|   IBIS model for TI tms320c6670 DSP
[IBIS Ver]   5.0
[Disclaimer]   Please be aware that in the absence of a written agreement
|   Texas Instruments(TI) assumes no liability for:
|   (1) The accuracy of the IBIS models provided to your company,
|   however, the IBIS model is compliant to industry standard
|   IQ Level 2a.  Refer to IBIS Quality Section below for
|   for full details.
|   (2) The proper functioning of these Models in your design
|   or for any resulting applications
|   (3) Infringement of patents, copyrights or intellectual
|   property rights resulting from your use of these
|   models.
|   TI provides IBIS Models as a service to our customers and
|   therefore reserves the right to limit distribution of the
|   Models.  The information is subject to change without notice.
[File Name]  tms320c6670_r1p11.ibs
[File Rev]   1.11
[Date]   16Feb2012
[Source]   Texas Instruments Incorporated
[Copyright]   Property of Texas Instruments Incorporated.
|   Unauthorized reproduction and/or distribution is strictly.
|   prohibited.
|   This product is protected under copyright law and trade
|   secret law as an unpublished work.
|   Created 2010,(C) Copyright 1999-2010,
|   Texas Instruments Incorporated., All Rights Reserved.
|   These commodities are under the U.S. Government
|   distribution license control. As such,they are not to be
|   re-exported without the prior approval of the U.S.
|   Department of Commerce.
[Notes]
   For SerDes simulations use Texas Instruments IBIS AMI models
   Some IV curves contain Non monotonic data points.
|   Model Generated by R.L.L.
|   **For SerDes simulations use Texas Instruments IBIS AMI models**
| Definitions:
|   NT   No termination
|   HT_TH_8mA   Half Termination Thevenin  [50 ohm] [100ohm to Vtt]
|   FT_TH_8mA   Full Termination Thevenin  [50 ohm] [50ohm to Vtt]
|   HT_TH_9mA   Half Termination Thevenin  [45 ohm] [90ohm to Vtt]
|   FT_TH_9mA   Full Termination Thevenin  [45 ohm] [45ohm to Vtt]
|   HT_TH_10mA   Half Termination Thevenin  [40 ohm] [80ohm to Vtt]
|   FT_TH_10mA   Full Termination Thevenin  [40 ohm] [40ohm to Vtt]
| Slew Rate Definitions:
| The Driver Slew Rate is defined by the value of the slew rate pins
|   DDRSLRATE1  DDRSLRATE0
|   FASTEST Slew Rate :   SR1 0;   SR0 0
|   FAST Slew Rate   :   SR1 0;   SR0 1
|   SLOW Slew Rate   :   SR1 1;   SR0 0
|   SLOWEST Slew Rate :   SR1 1;   SR0 1
| To choose the correct model, determine the settings of the DDRSLRATE[1:0] pins.
| Look for the keyword from the tables above to select the proper models.  For
| example; with the recommended 45.3ohm resistor connected to the PTV15 pin the
| drive strength of 9ma would be obtained "9MA_FT9MA". If the DDRSLRATE1 pin is
| pulled high and the DDRSLRATE0 pin is pulled low the slew rate (from the table
| above) would be "SLOW".  For this example the model needed for the address and
| control pins would be CSCDVG_SLOW_9MA, the data and DQM pins would be
| CSCDVG_SLOW_9MA_FT9MA and the DQS pins would be CSCDDVG_SLOW_9MA_FT9MA_N and
| CSCDDVG_SLOW_9MA_FT9MA_P.
|   Revision History
|   GERNERAL COMMENT: All IBIS Quality Notes below reflect latest release
|   and version of IBIS File
|   Revision 1.11 --16Feb 2012
|   -Corrected slew rate settings for fast and slow
|   -Added additional comments in the notes section
|   Revision 1.10 --14Oct 2011
|   -Updated model selectors
|   Revision 1.9 --12Oct 2011
|   -Corrected ACC_OUT & CLK_OUT descriptions
|   Revision 1.8 --29Sept 2011
|   -Corrected cell call error, removed Diff conflicting cells
|   Revision 1.7 --22Sept 2011
|   -Added submodels for bshtltcscddvg and bshtltcscdvg
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[Component] tms320c6670
[Manufacturer] Texas Instruments
[Package Model] 6670
[Package]
|Variable   Typ   Min   Max
R_pkg   1.0013   0.15483   2.0653
L_pkg   2.89689nH  0.94768nH   5.3815nH
C_pkg   1.63791pF  0.87102pF   2.5609pF
[Pin]   signal_name   model_name
A1   VSS   GND   |   GND
A10   DDRDQM4   DM   |   bshtltcscdvg
A11   DVDD15   POWER   |   POWER
A12   DDRCLKOUTP0   CLK_OUT   |   bshtltcscdvg
A13   DDRBA0   ACC_OUT   |   bshtltcscdvg
A14   DDRA00   ACC_OUT   |   bshtltcscdvg
A15   DDRA04   ACC_OUT   |   bshtltcscdvg
A16   DDRCLKOUTP1   CLK_OUT   |   bshtltcscdvg
A17   DVDD15   POWER   |   POWER
A18   DDRCB07   DQ   |   bshtltcscdvg
A19   DDRDQS8P   DQS   |   bshtltcscddvg
A2   DVDD15   POWER   |   POWER
A20   DDRDQM8   DM   |   bshtltcscdvg
A21   DDRDQS3P   DQS   |   bshtltcscddvg
A22   DDRDQM3   DM   |   bshtltcscdvg
A23   DDRD20   DQ   |   bshtltcscdvg
A24   DDRDQS2P   DQS   |   bshtltcscddvg
A25   DDRDQM2   DM   |   bshtltcscdvg
A26   DDRD15   DQ   |   bshtltcscdvg
A27   DDRDQS1P   DQS   |   bshtltcscddvg
A28   DVDD15   POWER   |   POWER
A29   VSS   GND   |   GND
A3   DDRDQS6N   DQS   |   bshtltcscddvg
A4   DDRD51   DQ   |   bshtltcscdvg
A5   DDRD49   DQ   |   bshtltcscdvg
A6   DDRDQS5N   DQS   |   bshtltcscddvg
A7   DDRD40   DQ   |   bshtltcscd
A8   DDRDQM5   DM   |   bshtltcscdvg
A9   DDRDQS4P   DQS   |   bshtltcscddvg
AA1   MCMTXPMDAT   bc1850cghypbfb   |   bc1850cghypbfb
AA10   CVDD   POWER   |   POWER
AA11   VSS   GND   |   GND
AA12   CVDD   POWER   |   POWER
AA13   VSS   GND   |   GND
AA14   CVDD   POWER   |   POWER
AA15   VSS   GND   |   GND
AA16   CVDD   POWER   |   POWER
AA17   VSS   GND   |   GND
AA18   CVDD   POWER   |   POWER
AA19   VSS   GND   |   GND
AA2   MCMTXPMCLK   bc1850cghypbfb   |   bc1850cghypbfb
AA20   CVDD   POWER   |   POWER
AA21   VSS   GND   |   GND
AA22   CVDD   POWER   |   POWER
AA23   VSS   GND   |   GND
AA24   RSV18   NC   |   NC
AA25   VSS   GND   |   GND
AA26   SYSCLKOUT   bc1850cghypbfb   |   bc1850cghypbfb
AA27   RADSYNC   bc1850cghypbfb   |   bc1850cghypbfb
AA28   RP1CLKN   ilvds18g   |   ilvds18g
AA29   RP1FBN   ilvds18g   |   ilvds18g
AA3   MCMRXPMCLK   bc1850cghypbfb   |   bc1850cghypbfb
AA4   VCNTL2   bi2c18gfz   |   bi2c18gfz
AA5   VSS   GND   |   GND
AA6   VSS   GND   |   GND
AA7   VSS   GND   |   GND
AA8   CVDD   POWER   |   POWER
AA9   VSS   GND   |   GND
AB1   VCNTL3   bi2c18gfz   |   bi2c18gfz
AB10   VSS   GND   |   GND
AB11   VSS   GND   |   GND
AB12   VSS   GND   |   GND
AB13   VSS   GND   |   GND
AB14   VSS   GND   |   GND
AB15   AVDDA3   POWER   |   POWER
AB16   VSS   GND   |   GND
AB17   DVDD18   POWER   |   POWER
AB18   VSS   GND   |   GND
AB19   DVDD18   POWER   |   POWER
AB2   VSS   GND   |   GND
AB20   VSS   GND   |   GND
AB21   DVDD18   POWER   |   POWER
AB22   VSS   GND   |   GND
AB23   CVDD   POWER   |   POWER
AB24   VSS   GND   |   GND
AB25   CORECLKSEL   bc1850cghypbfb   |   bc1850cghypbfb
AB26   RSV20   NC   |   NC
AB27   PHYSYNC   bc1850cghypbfb   |   bc1850cghypbfb
AB28   ALTCORECLKN   iclkrx10g   |   iclkrx10g
AB29   ALTCORECLKP   iclkrx10g   |   iclkrx10g
AB3   VCNTL1   bi2c18gfz   |   bi2c18gfz
AB4   VCNTL0   bi2c18gfz   |   bi2c18gfz
AB5   DVDD18   POWER   |   POWER
AB6   VSS   GND   |   GND
AB7   VSS   GND   |   GND
AB8   VSS   GND   |   GND
AB9   VSS   GND   |   GND
AC1   VSS   GND   |   GND
AC10   VDDT2   POWER   |   POWER
AC11   VSS   GND   |   GND
AC12   VDDT2   POWER   |   POWER
AC13   VSS   GND   |   GND
AC14   VDDT2   POWER   |   POWER
AC15   VSS   GND   |   GND
AC16   CORESEL1   bc1850cghypbfb   |   bc1850cghypbfb
AC17   SCL   bi2c18gfz   |   bi2c18gfz
AC18   HOUT   bc1840dghypbfb   |   bc1840dghypbfb
AC19   PORz   ihhv18g   |   RESET
AC2   DVDD18   POWER   |   POWER
AC20   LRESETNMIENz   bc1850cghypbfb   |   bc1850cghypbfb
AC21   BOOTCOMPLETE   bc1850cghypbfb   |   bc1850cghypbfb
AC22   RSV13   NC   |   NC
AC23   RSV03   NC   |   NC
AC24   RESETz   ic18ghypbfb   |   ic18ghypbfb
AC25   NMIz   bc1850cghypbfb   |   bc1850cghypbfb
AC26   TMS   ic18ghypbfb   |   ic18ghypbfb
AC27   TDO   bc1840dghypbfb   |   bc1840dghypbfb
AC28   SYSCLKN   iclkrx10g   |   iclkrx10g
AC29   SYSCLKP   iclkrx10g   |   iclkrx10g
AC3   VSS   GND   |   GND
AC4   DVDD18   POWER   |   POWER
AC5   VSS   GND   |   GND
AC6   VDDT2   POWER   |   POWER
AC7   VSS   GND   |   GND
AC8   VDDT2   POWER   |   POWER
AC9   VSS   GND   |   GND
AD1   CVDD1   POWER   |   POWER
AD10   VSS   GND   |   GND
AD11   VDDT2   POWER   |   POWER
AD12   VSS   GND   |   GND
AD13   VDDT2   POWER   |   POWER
AD14   VSS   GND   |   GND
AD15   CORESEL2   bc1850cghypbfb   |   bc1850cghypbfb
AD16   RSV23   NC   |   NC
AD17   SDA   bi2c18gfz   |   bi2c18gfz
AD18   RESETSTATz   bc1850cghypbfb   |   bc1850cghypbfb
AD19   GPIO02   bc1840dghypbfb   |   bc1840dghypbfb
AD2   VSS   GND   |   GND
AD20   GPIO11   bc1840dghypbfb   |   bc1840dghypbfb
AD21   GPIO15   bc1840dghypbfb   |   bc1840dghypbfb
AD22   RSV12   NC   |   NC
AD23   PACLKSEL   bc1840dghypbfb   |   bc1840dghypbfb
AD24   VSS   GND   |   GND
AD25   EMU05   bc1840dghypbfb   |   bc1840dghypbfb
AD26   TRSTz   ic18ghypbfb   |   ic18ghypbfb
AD27   VSS   GND   |   GND
AD28   TDI   ic18ghypbfb   |   ic18ghypbfb
AD29   TCK   ic18ghypbfb   |   ic18ghypbfb
AD3   CVDD1   POWER   |   POWER
AD4   VSS   GND   |   GND
AD5   VDDT2   POWER   |   POWER
AD6   VSS   GND   |   GND
AD7   VDDT2   POWER   |   POWER
AD8   VSS   GND   |   GND
AD9   VDDT2   POWER   |   POWER
AE1   VSS   GND   |   GND
AE10   VDDT2   POWER   |   POWER
AE11   VDDR4   POWER   |   POWER
AE12   VDDT2   POWER   |   POWER
AE13   VSS   GND   |   GND
AE14   RSV16   NC   |   NC
AE15   VDDR2   POWER   |   POWER
AE16   RSV22   NC   |   NC
AE17   EXTFRAMEEVENT   bc1850cghypbfb   |   bc1850cghypbfb
AE18   GPIO05   bc1840dghypbfb   |   bc1840dghypbfb
AE19   GPIO03   bc1840dghypbfb   |   bc1840dghypbfb
AE2   CVDD1   POWER   |   POWER
AE20   GPIO12   bc1840dghypbfb   |   bc1840dghypbfb
AE21   GPIO09   bc1840dghypbfb   |   bc1840dghypbfb
AE22   LRESETz   bc1850cghypbfb   |   bc1850cghypbfb
AE23   RESETFULLz   ic18ghypbfb   |   ic18ghypbfb
AE24   DVDD18   POWER   |   POWER
AE25   EMU07   bc1840dghypbfb   |   bc1840dghypbfb
AE26   EMU04   bc1840dghypbfb   |   bc1840dghypbfb
AE27   DVDD18   POWER   |   POWER
AE28   EMU02   bc1840dghypbfb   |   bc1840dghypbfb
AE29   EMU00   bc1840dghypbfb   |   bc1840dghypbfb
AE3   VSS   GND   |   GND
AE4   VDDT2   POWER   |   POWER
AE5   RSV17   NC   |   NC
AE6   VDDR3   POWER   |   POWER
AE7   VSS   GND   |   GND
AE8   RSV15   NC   |   NC
AE9   VSS   GND   |   GND
AF1   CVDD1   POWER   |   POWER
AF10   RIOTXP1   NC   |   NC
AF11   VSS   GND   |   GND
AF12   PCIETXN1   NC   |   NC
AF13   PCIETXP1   NC   |   NC
AF14   VSS   GND   |   GND
AF15   VSS   GND   |   GND
AF16   MDCLK   bc1840dghypbfb   |   bc1840dghypbfb
AF17   RSV25   NC   |   NC
AF18   GPIO04   bc1840dghypbfb   |   bc1840dghypbfb
AF19   DVDD18   POWER   |   POWER
AF2   VSS   GND   |   GND
AF20   VSS   GND   |   GND
AF21   GPIO13   bc1840dghypbfb   |   bc1840dghypbfb
AF22   DVDD18   POWER   |   POWER
AF23   TIMO1   bc1850cghypbfb   |   bc1850cghypbfb
AF24   UARTRXD   bc1850cghypbfb   |   bc1850cghypbfb
AF25   EMU06   bc1840dghypbfb   |   bc1840dghypbfb
AF26   EMU10   bc1840dghypbfb   |   bc1840dghypbfb
AF27   EMU08   bc1840dghypbfb   |   bc1840dghypbfb
AF28   EMU03   bc1840dghypbfb   |   bc1840dghypbfb
AF29   EMU01   bc1840dghypbfb   |   bc1840dghypbfb
AF3   SGMII0TXN   NC   |   NC
AF4   SGMII0TXP   NC   |   NC
AF5   VSS   GND   |   GND
AF6   RIOTXN3   NC   |   NC
AF7   RIOTXP3   NC   |   NC
AF8   VSS   GND   |   GND
AF9   RIOTXN1   NC   |   NC
AG1   VSS   GND   |   GND
AG10   RIOTXP0   NC   |   NC
AG11   RIOTXN0   NC   |   NC
AG12   VSS   GND   |   GND
AG13   PCIETXP0   NC   |   NC
AG14   PCIETXN0   NC   |   NC
AG15   VSS   GND   |   GND
AG16   MDIO   bc1850cghypbfb   |   bc1850cghypbfb
AG17   RSV24   NC   |   NC
AG18   GPIO01   bc1840dghypbfb   |   bc1840dghypbfb
AG19   GPIO10   bc1840dghypbfb   |   bc1840dghypbfb
AG2   CVDD1   POWER   |   POWER
AG20   GPIO06   bc1840dghypbfb   |   bc1840dghypbfb
AG21   SPICLK   bc1850cghypbfb   |   bc1850cghypbfb
AG22   VSS   GND   |   GND
AG23   TIMI1   bc1850cghypbfb   |   bc1850cghypbfb
AG24   UARTRTS   bc1850cghypbfb   |   bc1850cghypbfb
AG25   EMU13   bc1840dghypbfb   |   bc1840dghypbfb
AG26   VSS   GND   |   GND
AG27   EMU12   bc1840dghypbfb   |   bc1840dghypbfb
AG28   EMU11   bc1840dghypbfb   |   bc1840dghypbfb
AG29   EMU09   bc1840dghypbfb   |   bc1840dghypbfb
AG3   VSS   GND   |   GND
AG4   SGMII1TXN   NC   |   NC
AG5   SGMII1TXP   NC   |   NC
AG6   VSS   GND   |   GND
AG7   RIOTXN2   NC   |   NC
AG8   RIOTXP2   NC   |   NC
AG9   VSS   GND   |   GND
AH1   CVDD1   POWER   |   POWER
AH10   RIORXN1   NC   |   NC
AH11   VSS   GND   |   GND
AH12   PCIERXN1   NC   |   NC
AH13   PCIERXP1   NC   |   NC
AH14   VSS   GND   |   GND
AH15   CORESEL0   bc1850cghypbfb   |   bc1850cghypbfb
AH16   SRIOSGMIICLKN   iclkrx10g   |   iclkrx10g
AH17   PCIECLKP   iclkrx10g   |   iclkrx10g
AH18   PASSCLKN   iclkrx10g   |   iclkrx10g
AH19   GPIO07   bc1840dghypbfb   |   bc1840dghypbfb
AH2   VSS   GND   |   GND
AH20   GPIO14   bc1840dghypbfb   |   bc1840dghypbfb
AH21   SPISCS0   bc1850cghypbfb   |   bc1850cghypbfb
AH22   SPIDIN   bc1850cghypbfb   |   bc1850cghypbfb
AH23   TIMO0   bc1850cghypbfb   |   bc1850cghypbfb
AH24   UARTCTS   bc1850cghypbfb   |   bc1850cghypbfb
AH25   EMU18   bc1840dghypbfb   |   bc1840dghypbfb
AH26   DVDD18   POWER   |   POWER
AH27   EMU16   bc1840dghypbfb   |   bc1840dghypbfb
AH28   EMU14   bc1840dghypbfb   |   bc1840dghypbfb
AH29   DVDD18   POWER   |   POWER
AH3   SGMII0RXN   NC   |   NC
AH4   SGMII0RXP   NC   |   NC
AH5   VSS   GND   |   GND
AH6   RIORXN3   NC   |   NC
AH7   RIORXP3   NC   |   NC
AH8   VSS   GND   |   GND
AH9   RIORXP1   NC   |   NC
AJ1   VSS   GND   |   GND
AJ10   RIORXP0   NC   |   NC
AJ11   RIORXN0   NC   |   NC
AJ12   VSS   GND   |   GND
AJ13   PCIERXP0   NC   |   NC
AJ14   PCIERXN0   NC   |   NC
AJ15   VSS   GND   |   GND
AJ16   SRIOSGMIICLKP   iclkrx10g   |   iclkrx10g
AJ17   PCIECLKN   iclkrx10g   |   iclkrx10g
AJ18   PASSCLKP   iclkrx10g   |   iclkrx10g
AJ19   GPIO08   bc1840dghypbfb   |   bc1840dghypbfb
AJ2   CVDD1   POWER   |   POWER
AJ20   GPIO00   bc1840dghypbfb   |   bc1840dghypbfb
AJ21   SPIDOUT   bc1850cghypbfb   |   bc1850cghypbfb
AJ22   SPISCS1   bc1850cghypbfb   |   bc1850cghypbfb
AJ23   TIMI0   bc1850cghypbfb   |   bc1850cghypbfb
AJ24   UARTTXD   bc1850cghypbfb   |   bc1850cghypbfb
AJ25   RSV01   NC   |   NC
AJ26   EMU17   bc1840dghypbfb   |   bc1840dghypbfb
AJ27   EMU15   bc1840dghypbfb   |   bc1840dghypbfb
AJ28   DVDD18   POWER   |   POWER
AJ29   VSS   GND   |   GND
AJ3   VSS   GND   |   GND
AJ4   SGMII1RXN   NC   |   NC
AJ5   SGMII1RXP   NC   |   NC
AJ6   VSS   GND   |   GND
AJ7   RIORXN2   NC   |   NC
AJ8   RIORXP2   NC   |   NC
AJ9   VSS   GND   |   GND
B1   DVDD15   POWER   |   POWER
B10   DDRD34   DQ   |   bshtltcscdvg
B11   VSS   GND   |   GND
B12   DDRCLKOUTN0   CLK_OUT   |   bshtltcscdvg
B13   DDRBA1   ACC_OUT   |   bshtltcscdvg
B14   DDRA01   ACC_OUT   |   bshtltcscdvg
B15   DDRA06   ACC_OUT   |   bshtltcscdvg
B16   DDRCLKOUTN1   CLK_OUT   |   bshtltcscdvg
B17   VSS   GND   |   GND
B18   DDRCB06   DQ   |   bshtltcscdvg
B19   DDRDQS8N   DQS   |   bshtltcscddvg
B2   DDRDQM7   DM   |   bshtltcscdvg
B20   DDRCB03   DQ   |   bshtltcscdvg
B21   DDRDQS3N   DQS   |   bshtltcscddvg
B22   DDRD30   DQ   |   bshtltcscdvg
B23   DDRD21   DQ   |   bshtltcscdvg
B24   DDRDQS2N   DQS   |   bshtltcscddvg
B25   VSS   GND   |   GND
B26   DDRD14   DQ   |   bshtltcscdvg
B27   DDRDQS1N   DQS   |   bshtltcscddvg
B28   DDRD05   DQ   |   bshtltcscdvg
B29   DVDD15   POWER   |   POWER
B3   DDRDQS6P   DQS   |   bshtltcscddvg
B4   DDRD50   DQ   |   bshtltcscdvg
B5   DDRDQM6   DM   |   bshtltcscdvg
B6   DDRDQS5P   DQS   |   bshtltcscddvg
B7   DDRD44   DQ   |   bshtltcscdvg
B8   DDRD38   DQ   |   bshtltcscdvg
B9   DDRDQS4N   DQS   |   bshtltcscddvg
C1   DDRDQS7N   DQS   |   bshtltcscddvg
C10   DDRRASz   ACC_OUT   |   bshtltcscdvg
C11   DDRCE0z   ACC_OUT   |   bshtltcscdvg
C12   DDRCE1z   ACC_OUT   |   bshtltcscdvg
C13   DDRBA2   ACC_OUT   |   bshtltcscdvg
C14   DVDD15   POWER   |   POWER
C15   DDRA05   ACC_OUT   |   bshtltcscdvg
C16   DDRA13   ACC_OUT   |   bshtltcscdvg
C17   DDRA15   ACC_OUT   |   bshtltcscdvg
C18   DDRCB05   DQ   |   bshtltcscdvg
C19   DDRCB04   DQ   |   bshtltcscdvg
C2   DDRD59   DQ   |   bshtltcscdvg
C20   DDRCB01   DQ   |   bshtltcscdvg
C21   DDRD29   DQ   |   bshtltcscdvg
C22   DDRD31   DQ   |   bshtltcscdvg
C23   VSS   GND   |   GND
C24   DDRD22   DQ   |   bshtltcscdvg
C25   DVDD15   POWER   |   POWER
C26   DDRD13   DQ   |   bshtltcscdvg
C27   DDRDQM1   DM   |   bshtltcscdvg
C28   DDRDQS0P   DQS   |   bshtltcscddvg
C29   DDRDQS0N   DQS   |   bshtltcscddvg
C3   DDRD55   DQ   |   bshtltcscdvg
C4   DDRD54   DQ   |   bshtltcscdvg
C5   DDRD48   DQ   |   bshtltcscdvg
C6   DDRD47   DQ   |   bshtltcscdvg
C7   DDRD43   DQ   |   bshtltcscdvg
C8   VSS   GND   |   GND
C9   DDRD37   DQ   |   bshtltcscdvg
D1   DDRDQS7P   DQS   |   bshtltcscddvg
D10   DDRD33   DQ   |   bshtltcscdvg
D11   DDRCKE0   ACC_OUT   |   bshtltcscdvg
D12   DDRCASz   ACC_OUT   |   bshtltcscdvg
D13   DDRODT0   ACC_OUT   |   bshtltcscdvg
D14   VSS   GND   |   GND
D15   DDRA07   ACC_OUT   |   bshtltcscdvg
D16   DDRA11   ACC_OUT   |   bshtltcscdvg
D17   DDRA14   ACC_OUT   |   bshtltcscdvg
D18   VSS   GND   |   GND
D19   DDRCB02   DQ   |   bshtltcscdvg
D2   DDRD57   DQ   |   bshtltcscdvg
D20   DVDD15   POWER   |   POWER
D21   DDRD24   DQ   |   bshtltcscdvg
D22   DDRD28   DQ   |   bshtltcscdvg
D23   DVDD15   POWER   |   POWER
D24   DDRD18   DQ   |   bshtltcscdvg
D25   DDRD11   DQ   |   bshtltcscdvg
D26   DDRD12   DQ   |   bshtltcscdvg
D27   DDRD04   DQ   |   bshtltcscdvg
D28   DDRD03   DQ   |   bshtltcscdvg
D29   DDRD01   DQ   |   bshtltcscdvg
D3   VSS   GND   |   GND
D4   DDRD52   DQ   |   bshtltcscdvg
D5   DVDD15   POWER   |   POWER
D6   DDRD46   DQ   |   bshtltcscdvg
D7   DDRD41   DQ   |   bshtltcscdvg
D8   DVDD15   POWER   |   POWER
D9   DDRD35   DQ   |   bshtltcscdvg
E1   DDRD62   DQ   |   bshtltcscdvg
E10   DDRD32   DQ   |   bshtltcscdvg
E11   DDRRESETz   ACC_OUT   |   bshtltcscdvg
E12   DDRWEz   ACC_OUT   |   bshtltcscdvg
E13   DDRODT1   ACC_OUT   |   bshtltcscdvg
E14   VREFSSTL   NC   |   NC
E15   DDRA09   ACC_OUT   |   bshtltcscdvg
E16   DDRA10   ACC_OUT   |   bshtltcscdvg
E17   DDRA12   ACC_OUT   |   bshtltcscdvg
E18   DDRCKE1   ACC_OUT   |   bshtltcscdvg
E19   DDRCB00   DQ   |   bshtltcscdvg
E2   DDRD58   DQ   |   bshtltcscdvg
E20   VSS   GND   |   GND
E21   DDRD26   DQ   |   bshtltcscdvg
E22   DDRD23   DQ   |   bshtltcscdvg
E23   DDRD19   DQ   |   bshtltcscdvg
E24   DDRD09   DQ   |   bshtltcscdvg
E25   DDRD10   DQ   |   bshtltcscdvg
E26   DDRD06   DQ   |   bshtltcscdvg
E27   DDRD02   DQ   |   bshtltcscdvg
E28   DDRD00   DQ   |   bshtltcscdvg
E29   DDRDQM0   DM   |   bshtltcscdvg
E3   DVDD15   POWER   |   POWER
E4   DDRD53   DQ   |   bshtltcscdvg
E5   VSS   GND   |   GND
E6   DDRD45   DQ   |   bshtltcscdvg
E7   DDRD42   DQ   |   bshtltcscdvg
E8   DDRD39   DQ   |   bshtltcscdvg
E9   DDRD36   DQ   |   bshtltcscdvg
F1   DDRD63   DQ   |   bshtltcscdvg
F10   VSS   GND   |   GND
F11   DVDD15   POWER   |   POWER
F12   VSS   GND   |   GND
F13   DDRA03   ACC_OUT   |   bshtltcscdvg
F14   DDRA02   ACC_OUT   |   bshtltcscdvg
F15   DDRA08   ACC_OUT   |   bshtltcscdvg
F16   VSS   GND   |   GND
F17   DVDD15   POWER   |   POWER
F18   VSS   GND   |   GND
F19   DVDD15   POWER   |   POWER
F2   DDRD60   DQ   |   bshtltcscdvg
F20   DDRD25   DQ   |   bshtltcscdvg
F21   DDRD27   DQ   |   bshtltcscdvg
F22   DDRD17   DQ   |   bshtltcscdvg
F23   DDRD16   DQ   |   bshtltcscdvg
F24   DDRD08   DQ   |   bshtltcscdvg
F25   DDRD07   DQ   |   bshtltcscdvg
F26   VSS   GND   |   GND
F27   DVDD15   POWER   |   POWER
F28   VSS   GND   |   GND
F29   VSS   GND   |   GND
F3   DDRD61   DQ   |   bshtltcscdvg
F4   DDRD56   DQ   |   bshtltcscdvg
F5   DVDD15   POWER   |   POWER
F6   VSS   GND   |   GND
F7   DVDD15   POWER   |   POWER
F8   VSS   GND   |   GND
F9   DVDD15   POWER   |   POWER
G1   VSS   GND   |   GND
G10   DVDD15   POWER   |   POWER
G11   VSS   GND   |   GND
G12   DVDD15   POWER   |   POWER
G13   VSS   GND   |   GND
G14   DVDD15   POWER   |   POWER
G15   VSS   GND   |   GND
G16   DVDD15   POWER   |   POWER
G17   VSS   GND   |   GND
G18   DVDD15   POWER   |   POWER
G19   VSS   GND   |   GND
G2   DVDD15   POWER   |   POWER
G20   DVDD15   POWER   |   POWER
G21   VSS   GND   |   GND
G22   DVDD15   POWER   |   POWER
G23   VSS   GND   |   GND
G24   DVDD15   POWER   |   POWER
G25   VSS   GND   |   GND
G26   RSV21   NC   |   NC
G27   RSV19   NC   |   NC
G28   DVDD18   POWER   |   POWER
G29   DDRCLKP   iclkrx10g   |   iclkrx10g
G3   VSS   GND   |   GND
G4   DVDD15   POWER   |   POWER
G5   VSS   GND   |   GND
G6   CVDD1   POWER   |   POWER
G7   VSS   GND   |   GND
G8   DVDD15   POWER   |   POWER
G9   VSS   GND   |   GND
H1   CVDD1   POWER   |   POWER
H10   VSS   GND   |   GND
H11   CVDD   POWER   |   POWER
H12   VSS   GND   |   GND
H13   CVDD   POWER   |   POWER
H14   VSS   GND   |   GND
H15   CVDD   POWER   |   POWER
H16   VSS   GND   |   GND
H17   CVDD   POWER   |   POWER
H18   VSS   GND   |   GND
H19   CVDD   POWER   |   POWER
H2   VSS   GND   |   GND
H20   VSS   GND   |   GND
H21   CVDD   POWER   |   POWER
H22   VSS   GND   |   GND
H23   RSV10   NC   |   NC
H24   PTV15   NC   |   NC
H25   DVDD18   POWER   |   POWER
H26   DDRSLRATE1   bc1850cghypbfb   |   bc1850cghypbfb
H27   DDRSLRATE0   bc1850cghypbfb   |   bc1850cghypbfb
H28   RSV07   NC   |   NC
H29   DDRCLKN   iclkrx10g   |   iclkrx10g
H3   CVDD1   POWER   |   POWER
H4   VSS   GND   |   GND
H5   CVDD1   POWER   |   POWER
H6   VSS   GND   |   GND
H7   CVDD1   POWER   |   POWER
H8   VSS   GND   |   GND
H9   CVDD1   POWER   |   POWER
J1   VSS   GND   |   GND
J10   CVDD1   POWER   |   POWER
J11   VSS   GND   |   GND
J12   CVDD   POWER   |   POWER
J13   VSS   GND   |   GND
J14   CVDD1   POWER   |   POWER
J15   VSS   GND   |   GND
J16   CVDD1   POWER   |   POWER
J17   VSS   GND   |   GND
J18   CVDD   POWER   |   POWER
J19   VSS   GND   |   GND
J2   CVDD1   POWER   |   POWER
J20   CVDD1   POWER   |   POWER
J21   VSS   GND   |   GND
J22   CVDD1   POWER   |   POWER
J23   RSV11   NC   |   NC
J24   RSV08   NC   |   NC
J25   RSV09   NC   |   NC
J26   AVDDA2   POWER   |   POWER
J27   VSS   GND   |   GND
J28   RSV06   NC   |   NC
J29   VSS   GND   |   GND
J3   VSS   GND   |   GND
J4   CVDD1   POWER   |   POWER
J5   VSS   GND   |   GND
J6   CVDD1   POWER   |   POWER
J7   VSS   GND   |   GND
J8   CVDD1   POWER   |   POWER
J9   VSS   GND   |   GND
K1   VSS   GND   |   GND
K10   VSS   GND   |   GND
K11   CVDD   POWER   |   POWER
K12   VSS   GND   |   GND
K13   CVDD1   POWER   |   POWER
K14   VSS   GND   |   GND
K15   CVDD1   POWER   |   POWER
K16   VSS   GND   |   GND
K17   CVDD1   POWER   |   POWER
K18   VSS   GND   |   GND
K19   CVDD   POWER   |   POWER
K2   VSS   GND   |   GND
K20   VSS   GND   |   GND
K21   CVDD1   POWER   |   POWER
K22   VSS   GND   |   GND
K23   RSV0B   NC   |   NC
K24   RSV0A   NC   |   NC
K25   VDDT3   POWER   |   POWER
K26   VSS   GND   |   GND
K27   AIFTXP1   NC   |   NC
K28   VSS   GND   |   GND
K29   AIFRXN1   NC   |   NC
K3   VSS   GND   |   GND
K4   VSS   GND   |   GND
K5   VSS   GND   |   GND
K6   VDDR1   POWER   |   POWER
K7   CVDD1   POWER   |   POWER
K8   VSS   GND   |   GND
K9   CVDD1   POWER   |   POWER
L1   MCMRXN2   NC   |   NC
L10   CVDD1   POWER   |   POWER
L11   VSS   GND   |   GND
L12   CVDD   POWER   |   POWER
L13   VSS   GND   |   GND
L14   CVDD1   POWER   |   POWER
L15   VSS   GND   |   GND
L16   CVDD1   POWER   |   POWER
L17   VSS   GND   |   GND
L18   CVDD   POWER   |   POWER
L19   VSS   GND   |   GND
L2   VSS   GND   |   GND
L20   CVDD1   POWER   |   POWER
L21   VSS   GND   |   GND
L22   CVDD1   POWER   |   POWER
L23   VSS   GND   |   GND
L24   VDDT3   POWER   |   POWER
L25   RSV27   NC   |   NC
L26   AIFTXN0   NC   |   NC
L27   AIFTXN1   NC   |   NC
L28   AIFRXN0   NC   |   NC
L29   AIFRXP1   NC   |   NC
L3   VSS   GND   |   GND
L4   MCMTXN2   NC   |   NC
L5   VSS   GND   |   GND
L6   VSS   GND   |   GND
L7   VSS   GND   |   GND
L8   CVDD1   POWER   |   POWER
L9   VSS   GND   |   GND
M1   MCMRXP2   NC   |   NC
M10   VSS   GND   |   GND
M11   CVDD   POWER   |   POWER
M12   VSS   GND   |   GND
M13   CVDD   POWER   |   POWER
M14   VSS   GND   |   GND
M15   CVDD   POWER   |   POWER
M16   VSS   GND   |   GND
M17   CVDD   POWER   |   POWER
M18   VSS   GND   |   GND
M19   CVDD   POWER   |   POWER
M2   MCMRXP3   NC   |   NC
M20   VSS   GND   |   GND
M21   CVDD1   POWER   |   POWER
M22   VSS   GND   |   GND
M23   VDDT3   POWER   |   POWER
M24   VSS   GND   |   GND
M25   VDDT3   POWER   |   POWER
M26   AIFTXP0   NC   |   NC
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|********************  DIFF PIN  *******************************
[Diff_pin]   inv_pin   vdiff  tdelay_typ  tdelay_min  tdelay_max
A12   B12   200mV   NA   NA   NA   || DDRCLKOUTP0 & DDRCLKOUTN0
A16   B16   200mV   NA   NA   NA   || DDRCLKOUTP1 & DDRCLKOUTN1
C28   C29   200mV   NA   NA   NA   || DDRDQS0P & DDRDQS0N
A27   B27   200mV   NA   NA   NA   || DDRDQS1P & DDRDQS1N
A24   B24   200mV   NA   NA   NA   || DDRDQS2P & DDRDQS2N
A21   B21   200mV   NA   NA   NA   || DDRDQS3P & DDRDQS3N
A9   B9   200mV   NA   NA   NA   || DDRDQS4P & DDRDQS4N
B6   A6   200mV   NA   NA   NA   || DDRDQS5P & DDRDQS5N
B3   A3   200mV   NA   NA   NA   || DDRDQS6P & DDRDQS6N
D1   C1   200mV   NA   NA   NA   || DDRDQS7P & DDRDQS7N
A19   B19   200mV   NA   NA   NA   || DDRDQS8P & DDRDQS8N
AB29   AB28   100mV   NA   NA   NA   || ALTCORECLKP ALTCORECLKN
G29   H29   NA   NA   NA   NA   || DDRCLKP & DDRCLKN
W1   W2   NA   NA   NA   NA   || MCMCLKP & MCMCLKN
V2   V1   50mV   NA   NA   NA   || MCMREFCLKOUTP & MCMREFCLKOUTN
AJ18   AH18   NA   NA   NA   NA   || PASSCLKP & PASSCLKN
AH17   AJ17   NA   NA   NA   NA   || PCIECLKP & PCIECLKN
AJ16   AH16   100mV   NA   NA   NA   || SRIOSGMIICLKP & SRIOSGMIICLKN
AC29   AC28   100mV   NA   NA   NA   || SYSCLKP & SYSCLKN
Y28   AA28   100mV   NA   NA   NA   || RP1CLKP & RP1CLKN
[Model Selector] ocml10g
|ocml10g   [30Jul2010 Revision 1.0]
ocml10g_0p9 Model operating at 0.9V nom VDDS
|ocml10g_0p9;
ocml10g_1   Model operating at 1V nom VDDS
|ocml10g_1;
[Model Selector] bc1840dghypbfb
|bc1840dghypbfb.ibs   [15July11 revision 1.0]
BC1840DGHYPBFB_WK_PD  Cell operated at 1.8(nom)
|IO in Rx mode with weak pulldown on in 1.8V mode
BC1840DGHYPBFB_WK_PU  Cell operated at 1.8(nom)
|IO in Rx mode with weak pullup on  in 1.8V mode
BC1840DGHYPBFB_DRIVER_MODE  Cell operated at 1.8(nom)
|Normal IO mode of operation at 1.8V VDDS
[Model Selector] bc1850cghypbfb
|bc1850cghypbfb.ibs [15July2011 revision 1.0]
BC1850CGHYPBFB_WK_PD  Cell operated at 1.8(nom)
|IO in Rx mode with weak pulldown on  in 1.8V mode
BC1850CGHYPBFB_WK_PU  Cell operated at 1.8(nom)
|IO in Rx mode with weak pullup on in 1.8V mode
BC1850CGHYPBFB_DRIVER_MODE  Cell operated at 1.8(nom)
|   DDR ACC
[Model Selector]   ACC_OUT
| bshtltcscdvg.ibs   [6 Sep 2011 Revision 1.6]
CSCDVG_SLOWEST_8MA   TX 50 ohms Slowest (SR0 1; SR1 1)
CSCDVG_SLOW_8MA   TX 50 ohms Slow (SR0 1; SR1 0)
CSCDVG_FAST_8MA   TX 50 ohms Fast (SR0 0; SR1 1)
CSCDVG_FASTEST_8MA   TX 50 ohms Fastest (SR0 0; SR1 0)
CSCDVG_SLOWEST_9MA   TX 45 ohms Slowest (SR0 1; SR1 1)
CSCDVG_SLOW_9MA   TX 45 ohms Slow (SR0 1; SR1 0)
CSCDVG_FAST_9MA   TX 45 ohms Fast (SR0 0; SR1 1)
CSCDVG_FASTEST_9MA   TX 45 ohms Fastest (SR0 0; SR1 0)
CSCDVG_SLOWEST_10MA   TX 40 ohms Slowest (SR0 1; SR1 1)
CSCDVG_SLOW_10MA   TX 40 ohms Slow (SR0 1; SR1 0)
CSCDVG_FAST_10MA   TX 40 ohms Fast (SR0 0; SR1 1)
CSCDVG_FASTEST_10MA   TX 40 ohms Fastest (SR0 0; SR1 0)
|   DDR CLOCK_OUT
[Model Selector]   CLK_OUT
| bshtltcscdvg.ibs   [6 Sep 2011 Revision 1.6]
CSCDVG_SLOWEST_8MA   TX 50 ohms Slowest (SR0 1; SR1 1)
CSCDVG_SLOW_8MA   TX 50 ohms Slow (SR0 1; SR1 0)
CSCDVG_FAST_8MA   TX 50 ohms Fast (SR0 0; SR1 1)
CSCDVG_FASTEST_8MA   TX 50 ohms Fastest (SR0 0; SR1 0)
CSCDVG_SLOWEST_9MA   TX 45 ohms Slowest (SR0 1; SR1 1)
CSCDVG_SLOW_9MA   TX 45 ohms Slow (SR0 1; SR1 0)
CSCDVG_FAST_9MA   TX 45 ohms Fast (SR0 0; SR1 1)
CSCDVG_FASTEST_9MA   TX 45 ohms Fastest (SR0 0; SR1 0)
CSCDVG_SLOWEST_10MA   TX 40 ohms Slowest (SR0 1; SR1 1)
CSCDVG_SLOW_10MA   TX 40 ohms Slow (SR0 1; SR1 0)
CSCDVG_FAST_10MA   TX 40 ohms Fast (SR0 0; SR1 1)
CSCDVG_FASTEST_10MA   TX 40 ohms Fastest (SR0 0; SR1 0)
|   DDR DQ
[Model Selector] DQ
| bshtltcscdvg.ibs   [6 Sep 2011 Revision 1.6]
CSCDVG_SLOWEST_8MA_HT8MA   TX 50ohms Slowest or RX mode: [100ohm to Vtt]
CSCDVG_SLOWEST_8MA_FT8MA   TX 50ohms Slowest or RX mode: [50ohm to Vtt]
CSCDVG_SLOWEST_8MA_NT   TX 50ohms Slowest or RX mode: [No ODT]
CSCDVG_SLOW_8MA_HT8MA   TX 50ohms Slow or RX mode: [100ohm to Vtt]
CSCDVG_SLOW_8MA_FT8MA   TX 50ohms Slow or RX mode: [50ohm to Vtt]
CSCDVG_SLOW_8MA_NT   TX 50ohms Slow or RX mode: [No ODT]
CSCDVG_FAST_8MA_HT8MA   TX 50ohms Fast or RX mode: [100ohm to Vtt]
CSCDVG_FAST_8MA_FT8MA   TX 50ohms Fast or RX mode: [50ohm to Vtt]
CSCDVG_FAST_8MA_NT   TX 50ohms Fast or RX mode: [No ODT]
CSCDVG_FASTEST_8MA_HT8MA   TX 50ohms Fastest or RX mode: [100ohm to Vtt]
CSCDVG_FASTEST_8MA_FT8MA   TX 50ohms Fastest or RX mode: [50ohm to Vtt]
CSCDVG_FASTEST_8MA_NT   TX 50ohms Fastest or RX mode: [No ODT]
CSCDVG_SLOWEST_9MA_HT9MA   TX 45ohms Slowest or RX mode: [90ohm to Vtt]
CSCDVG_SLOWEST_9MA_FT9MA   TX 45ohms Slowest or RX mode: [45ohm to Vtt]
CSCDVG_SLOWEST_9MA_NT   TX 45ohms Slowest or RX mode: [No ODT]
CSCDVG_SLOW_9MA_HT9MA   TX 45ohms Slow or RX mode: [90ohm to Vtt]
CSCDVG_SLOW_9MA_FT9MA   TX 45ohms Slow or RX mode: [45ohm to Vtt]
CSCDVG_SLOW_9MA_NT   TX 45ohms Slow or RX mode: [No ODT]
CSCDVG_FAST_9MA_HT9MA   TX 45ohms Fast or RX mode: [90ohm to Vtt]
CSCDVG_FAST_9MA_FT9MA   TX 45ohms Fast or RX mode: [45ohm to Vtt]
CSCDVG_FAST_9MA_NT   TX 45ohms Fast or RX mode: [No ODT]
CSCDVG_FASTEST_9MA_HT9MA   TX 45ohms Fastest or RX mode: [90ohm to Vtt]
CSCDVG_FASTEST_9MA_FT9MA   TX 45ohms Fastest or RX mode: [45ohm to Vtt]
CSCDVG_FASTEST_9MA_NT   TX 45ohms Fastest or RX mode: [No ODT]
CSCDVG_SLOWEST_10MA_HT10MA TX 40ohms Slowest or RX mode: [80ohm to Vtt]
CSCDVG_SLOWEST_10MA_FT10MA TX 40ohms Slowest or RX mode: [40ohm to Vtt]
CSCDVG_SLOWEST_10MA_NT   TX 40ohms Slowest or RX mode: [No ODT]
CSCDVG_SLOW_10MA_HT10MA   TX 40ohms Slow or RX mode: [80ohm to Vtt]
CSCDVG_SLOW_10MA_FT10MA   TX 40ohms Slow or RX mode: [40ohm to Vtt]
CSCDVG_SLOW_10MA_NT   TX 40ohms Slow or RX mode: [No ODT]
CSCDVG_FAST_10MA_HT10MA   TX 40ohms Fast or RX mode: [80ohm to Vtt]
CSCDVG_FAST_10MA_FT10MA   TX 40ohms Fast or RX mode: [40ohm to Vtt]
CSCDVG_FAST_10MA_NT   TX 40ohms Fast or RX mode: [No ODT]
CSCDVG_FASTEST_10MA_HT10MA TX 40ohms Fastest or RX mode: [80ohm to Vtt]
CSCDVG_FASTEST_10MA_FT10MA TX 40ohms Fastest or RX mode: [40ohm to Vtt]
CSCDVG_FASTEST_10MA_NT   TX 40ohms Fastest or RX mode: [No ODT]
|   DDR DQM
[Model Selector] DM
| bshtltcscdvg.ibs   [6 Sep 2011 Revision 1.6]
CSCDVG_SLOWEST_8MA_HT8MA   TX 50ohms Slowest or RX mode: [100ohm to Vtt]
CSCDVG_SLOWEST_8MA_FT8MA   TX 50ohms Slowest or RX mode: [50ohm to Vtt]
CSCDVG_SLOWEST_8MA_NT   TX 50ohms Slowest or RX mode: [No ODT]
CSCDVG_SLOW_8MA_HT8MA   TX 50ohms Slow or RX mode: [100ohm to Vtt]
CSCDVG_SLOW_8MA_FT8MA   TX 50ohms Slow or RX mode: [50ohm to Vtt]
CSCDVG_SLOW_8MA_NT   TX 50ohms Slow or RX mode: [No ODT]
CSCDVG_FAST_8MA_HT8MA   TX 50ohms Fast or RX mode: [100ohm to Vtt]
CSCDVG_FAST_8MA_FT8MA   TX 50ohms Fast or RX mode: [50ohm to Vtt]
CSCDVG_FAST_8MA_NT   TX 50ohms Fast or RX mode: [No ODT]
CSCDVG_FASTEST_8MA_HT8MA   TX 50ohms Fastest or RX mode: [100ohm to Vtt]
CSCDVG_FASTEST_8MA_FT8MA   TX 50ohms Fastest or RX mode: [50ohm to Vtt]
CSCDVG_FASTEST_8MA_NT   TX 50ohms Fastest or RX mode: [No ODT]
CSCDVG_SLOWEST_9MA_HT9MA   TX 45ohms Slowest or RX mode: [90ohm to Vtt]
CSCDVG_SLOWEST_9MA_FT9MA   TX 45ohms Slowest or RX mode: [45ohm to Vtt]
CSCDVG_SLOWEST_9MA_NT   TX 45ohms Slowest or RX mode: [No ODT]
CSCDVG_SLOW_9MA_HT9MA   TX 45ohms Slow or RX mode: [90ohm to Vtt]
CSCDVG_SLOW_9MA_FT9MA   TX 45ohms Slow or RX mode: [45ohm to Vtt]
CSCDVG_SLOW_9MA_NT   TX 45ohms Slow or RX mode: [No ODT]
CSCDVG_FAST_9MA_HT9MA   TX 45ohms Fast or RX mode: [90ohm to Vtt]
CSCDVG_FAST_9MA_FT9MA   TX 45ohms Fast or RX mode: [45ohm to Vtt]
CSCDVG_FAST_9MA_NT   TX 45ohms Fast or RX mode: [No ODT]
CSCDVG_FASTEST_9MA_HT9MA   TX 45ohms Fastest or RX mode: [90ohm to Vtt]
CSCDVG_FASTEST_9MA_FT9MA   TX 45ohms Fastest or RX mode: [45ohm to Vtt]
CSCDVG_FASTEST_9MA_NT   TX 45ohms Fastest or RX mode: [No ODT]
CSCDVG_SLOWEST_10MA_HT10MA TX 40ohms Slowest or RX mode: [80ohm to Vtt]
CSCDVG_SLOWEST_10MA_FT10MA TX 40ohms Slowest or RX mode: [40ohm to Vtt]
CSCDVG_SLOWEST_10MA_NT   TX 40ohms Slowest or RX mode: [No ODT]
CSCDVG_SLOW_10MA_HT10MA   TX 40ohms Slow or RX mode: [80ohm to Vtt]
CSCDVG_SLOW_10MA_FT10MA   TX 40ohms Slow or RX mode: [40ohm to Vtt]
CSCDVG_SLOW_10MA_NT   TX 40ohms Slow or RX mode: [No ODT]
CSCDVG_FAST_10MA_HT10MA   TX 40ohms Fast or RX mode: [80ohm to Vtt]
CSCDVG_FAST_10MA_FT10MA   TX 40ohms Fast or RX mode: [40ohm to Vtt]
CSCDVG_FAST_10MA_NT   TX 40ohms Fast or RX mode: [No ODT]
CSCDVG_FASTEST_10MA_HT10MA TX 40ohms Fastest or RX mode: [80ohm to Vtt]
CSCDVG_FASTEST_10MA_FT10MA TX 40ohms Fastest or RX mode: [40ohm to Vtt]
CSCDVG_FASTEST_10MA_NT   TX 40ohms Fastest or RX mode: [No ODT]
|   DDR DQS
| Negative Pad
[Model Selector] DQS
| bshtltcscddvg.ibs   [6 Sep 2011 Revision 1.6]
CSCDDVG_SLOWEST_8MA_HT8MA_N   TX 50ohms Slowest or RX mode: [100ohm to Vtt]
CSCDDVG_SLOWEST_8MA_FT8MA_N   TX 50ohms Slowest or RX mode: [50ohm to Vtt]
CSCDDVG_SLOWEST_8MA_NT_N   TX 50ohms Slowest or RX mode: [No ODT]
CSCDDVG_SLOW_8MA_HT8MA_N   TX 50ohms Slow or RX mode: [100ohm to Vtt]
CSCDDVG_SLOW_8MA_FT8MA_N   TX 50ohms Slow or RX mode: [50ohm to Vtt]
CSCDDVG_SLOW_8MA_NT_N   TX 50ohms Slow or RX mode: [No ODT]
CSCDDVG_FAST_8MA_HT8MA_N   TX 50ohms Fast or RX mode: [100ohm to Vtt]
CSCDDVG_FAST_8MA_FT8MA_N   TX 50ohms Fast or RX mode: [50ohm to Vtt]
CSCDDVG_FAST_8MA_NT_N   TX 50ohms Fast or RX mode: [No ODT]
CSCDDVG_FASTEST_8MA_HT8MA_N   TX 50ohms Fastest or RX mode: [90ohm to Vtt]
CSCDDVG_FASTEST_8MA_FT8MA_N   TX 50ohms Fastest or RX mode: [45ohm to Vtt]
CSCDDVG_FASTEST_8MA_NT_N   TX 50ohms Fastest or RX mode: [No ODT]
CSCDDVG_SLOWEST_9MA_HT9MA_N   TX 45ohms Slowest or RX mode: [90ohm to Vtt]
CSCDDVG_SLOWEST_9MA_FT9MA_N   TX 45ohms Slowest or RX mode: [45ohm to Vtt]
CSCDDVG_SLOWEST_9MA_NT_N   TX 45ohms Slowest or RX mode: [No ODT]
CSCDDVG_SLOW_9MA_HT9MA_N   TX 45ohms Slow or RX mode: [90ohm to Vtt]
CSCDDVG_SLOW_9MA_FT9MA_N   TX 45ohms Slow or RX mode: [45ohm to Vtt]
CSCDDVG_SLOW_9MA_NT_N   TX 45ohms Slow or RX mode: [No ODT]
CSCDDVG_FAST_9MA_HT9MA_N   TX 45ohms Fast or RX mode: [90ohm to Vtt]
CSCDDVG_FAST_9MA_FT9MA_N   TX 45ohms Fast or RX mode: [45ohm to Vtt]
CSCDDVG_FAST_9MA_NT_N   TX 45ohms Fast or RX mode: [No ODT]
CSCDDVG_FASTEST_9MA_HT9MA_N   TX 45ohms Fastest or RX mode: [90ohm to Vtt]
CSCDDVG_FASTEST_9MA_FT9MA_N   TX 45ohms Fastest or RX mode: [45ohm to Vtt]
CSCDDVG_FASTEST_9MA_NT_N   TX 45ohms Fastest or RX mode: [No ODT]
CSCDDVG_SLOWEST_10MA_HT10MA_N TX 40ohms Slowest or RX mode: [80ohm to Vtt]
CSCDDVG_SLOWEST_10MA_FT10MA_N TX 40ohms Slowest or RX mode: [40ohm to Vtt]
CSCDDVG_SLOWEST_10MA_NT_N   TX 40ohms Slowest or RX mode: [No ODT]
CSCDDVG_SLOW_10MA_HT10MA_N   TX 40ohms Slow or RX mode: [80ohm to Vtt]
CSCDDVG_SLOW_10MA_FT10MA_N   TX 40ohms Slow or RX mode: [40ohm to Vtt]
CSCDDVG_SLOW_10MA_NT_N   TX 40ohms Slow or RX mode: [No ODT]
CSCDDVG_FAST_10MA_HT10MA_N   TX 40ohms Fast or RX mode: [80ohm to Vtt]
CSCDDVG_FAST_10MA_FT10MA_N   TX 40ohms Fast or RX mode: [40ohm to Vtt]
CSCDDVG_FAST_10MA_NT_N   TX 40ohms Fast or RX mode: [No ODT]
CSCDDVG_FASTEST_10MA_HT10MA_N TX 40ohms Fastest or RX mode: [80ohm to Vtt]
CSCDDVG_FASTEST_10MA_FT10MA_N TX 40ohms Fastest or RX mode: [40ohm to Vtt]
CSCDDVG_FASTEST_10MA_NT_N   TX 40ohms Fastest or RX mode: [No ODT]
|   DDR DQS
| Positive Pad
CSCDDVG_SLOWEST_8MA_HT8MA_P   TX 50ohms Slowest or RX mode: [100ohm to Vtt]
CSCDDVG_SLOWEST_8MA_FT8MA_P   TX 50ohms Slowest or RX mode: [50ohm to Vtt]
CSCDDVG_SLOWEST_8MA_NT_P   TX 50ohms Slowest or RX mode: [No ODT]
CSCDDVG_SLOW_8MA_HT8MA_P   TX 50ohms Slow or RX mode: [100ohm to Vtt]
CSCDDVG_SLOW_8MA_FT8MA_P   TX 50ohms Slow or RX mode: [50ohm to Vtt]
CSCDDVG_SLOW_8MA_NT_P   TX 50ohms Slow or RX mode: [No ODT]
CSCDDVG_FAST_8MA_HT8MA_P   TX 50ohms Fast or RX mode: [100ohm to Vtt]
CSCDDVG_FAST_8MA_FT8MA_P   TX 50ohms Fast or RX mode: [50ohm to Vtt]
CSCDDVG_FAST_8MA_NT_P   TX 50ohms Fast or RX mode: [No ODT]
CSCDDVG_FASTEST_8MA_HT8MA_P   TX 50ohms Fastest or RX mode: [90ohm to Vtt]
CSCDDVG_FASTEST_8MA_FT8MA_P   TX 50ohms Fastest or RX mode: [45ohm to Vtt]
CSCDDVG_FASTEST_8MA_NT_P   TX 50ohms Fastest or RX mode: [No ODT]
CSCDDVG_SLOWEST_9MA_HT9MA_P   TX 45ohms Slowest or RX mode: [90ohm to Vtt]
CSCDDVG_SLOWEST_9MA_FT9MA_P   TX 45ohms Slowest or RX mode: [45ohm to Vtt]
CSCDDVG_SLOWEST_9MA_NT_P   TX 45ohms Slowest or RX mode: [No ODT]
CSCDDVG_SLOW_9MA_HT9MA_P   TX 45ohms Slow or RX mode: [90ohm to Vtt]
CSCDDVG_SLOW_9MA_FT9MA_P   TX 45ohms Slow or RX mode: [45ohm to Vtt]
CSCDDVG_SLOW_9MA_NT_P   TX 45ohms Slow or RX mode: [No ODT]
CSCDDVG_FAST_9MA_HT9MA_P   TX 45ohms Fast or RX mode: [90ohm to Vtt]
CSCDDVG_FAST_9MA_FT9MA_P   TX 45ohms Fast or RX mode: [45ohm to Vtt]
CSCDDVG_FAST_9MA_NT_P   TX 45ohms Fast or RX mode: [No ODT]
CSCDDVG_FASTEST_9MA_HT9MA_P   TX 45ohms Fastest or RX mode: [90ohm to Vtt]
CSCDDVG_FASTEST_9MA_FT9MA_P   TX 45ohms Fastest or RX mode: [45ohm to Vtt]
CSCDDVG_FASTEST_9MA_NT_P   TX 45ohms Fastest or RX mode: [No ODT]
CSCDDVG_SLOWEST_10MA_HT10MA_P TX 40ohms Slowest or RX mode: [80ohm to Vtt]
CSCDDVG_SLOWEST_10MA_FT10MA_P TX 40ohms Slowest or RX mode: [40ohm to Vtt]
CSCDDVG_SLOWEST_10MA_NT_P   TX 40ohms Slowest or RX mode: [No ODT]
CSCDDVG_SLOW_10MA_HT10MA_P   TX 40ohms Slow or RX mode: [80ohm to Vtt]
CSCDDVG_SLOW_10MA_FT10MA_P   TX 40ohms Slow or RX mode: [40ohm to Vtt]
CSCDDVG_SLOW_10MA_NT_P   TX 40ohms Slow or RX mode: [No ODT]
CSCDDVG_FAST_10MA_HT10MA_P   TX 40ohms Fast or RX mode: [80ohm to Vtt]
CSCDDVG_FAST_10MA_FT10MA_P   TX 40ohms Fast or RX mode: [40ohm to Vtt]
CSCDDVG_FAST_10MA_NT_P   TX 40ohms Fast or RX mode: [No ODT]
CSCDDVG_FASTEST_10MA_HT10MA_P TX 40ohms Fastest or RX mode: [80ohm to Vtt]
CSCDDVG_FASTEST_10MA_FT10MA_P TX 40ohms Fastest or RX mode: [40ohm to Vtt]
CSCDDVG_FASTEST_10MA_NT_P   TX 40ohms Fastest or RX mode: [No ODT]
[Model Selector] ic18ghypbfb
| ic18ghypbfb.ibs  [11July2011 revision 1.0]
IC18GHYPBFB_WK_PD_ON   Cell operated at 1.8(nom)
IC18GHYPBFB_WK_PU_ON   Cell operated at 1.8(nom)
IC18GHYPBFB_RX_MODE   Cell operated at 1.8(nom)
[Model Selector] ilvds18g
| ilvds18g.ibs  [08Jul11 revision 1.2]
ilvds18g_5P   Cell operated at 1.8(nom)
s_ilvds18g_5P   Cell operated at 1.8(nom)
[Model Selector] iclkrx10g
iclkrx10g_0p9 Cell operated at 0p9(nom)
| iclkrx10g_0p9.ibs  [08Jul11 revision 1.3]
s_iclkrx10g_0p9 Cell operated at 0p9(nom)
| iclkrx10g_0p9.ibs  [08Jul11 revision 1.3]
iclkrx10g_1 Cell operated at 1p0(nom)
| iclkrx10g_1.ibs  [08Jul11 revision 1.2]
s_iclkrx10g_1 Cell operated at 1p0(nom)
|   Package Model Definition
[Define Package Model]  6670
[Manufacturer]   Texas Instruments Incorporated
[OEM]   Texas Instruments Incorporated
[Description]   6670 pkg with all signals except SERDES
|   From Apache Design Solutions' PakSi-E result
|   Package model generated 11Jun10
[Number Of Pins]   336
[Pin Numbers]
U25  | 1 BGA-U25 RSV26
U29  | 2 BGA-U29 AIFRXP4
U26  | 3 BGA-U26 AIFTXN5
L25  | 4 BGA-L25 RSV27
L26  | 5 BGA-L26 AIFTXN0
M26  | 6 BGA-M26 AIFTXP0
L28  | 7 BGA-L28 AIFRXN0
M28  | 8 BGA-M28 AIFRXP0
L27  | 9 BGA-L27 AIFTXN1
K29  | 10 BGA-K29 AIFRXN1
L29  | 11 BGA-L29 AIFRXP1
R28  | 12 BGA-R28 AIFRXN2
P28  | 13 BGA-P28 AIFRXP2
P26  | 14 BGA-P26 AIFTXP2
P29  | 15 BGA-P29 AIFRXN3
N29  | 16 BGA-N29 AIFRXP3
T29  | 17 BGA-T29 AIFRXN4
U27  | 18 BGA-U27 AIFTXN4
U28  | 19 BGA-U28 AIFRXN5
V28  | 20 BGA-V28 AIFRXP5
V26  | 21 BGA-V26 AIFTXP5
P27  | 22 BGA-P27 AIFTXN3
R26  | 23 BGA-R26 AIFTXN2
Y28  | 24 BGA-Y28 RP1CLKP
K27  | 25 BGA-K27 AIFTXP1
N27  | 26 BGA-N27 AIFTXP3
T27  | 27 BGA-T27 AIFTXP4
AB28 | 28 BGA-AB28 ALTCORECLKN
AB29 | 29 BGA-AB29 ALTCORECLKP
AC28 | 30 BGA-AC28 SYSCLKN
AC21 | 31 BGA-AC21 BOOTCOMPLETE
AE23 | 32 BGA-AE23 RESETFULLZ
AC18 | 33 BGA-AC18 HOUT
AA24 | 34 BGA-AA24 RSV18
AB26 | 35 BGA-AB26 RSV20
AA26 | 36 BGA-AA26 SYSCLKOUT
AB25 | 37 BGA-AB25 CORECLKSEL
AA27 | 38 BGA-AA27 RADSYNC
W27  | 39 BGA-W27 RSV05
Y27  | 40 BGA-Y27 RSV04
AH15 | 41 BGA-AH15 CORESEL0
AG19 | 42 BGA-AG19 GPIO10
AD17 | 43 BGA-AD17 SDA
AC16 | 44 BGA-AC16 CORESEL1
AC17 | 45 BGA-AC17 SCL
AD15 | 46 BGA-AD15 CORESEL2
G27  | 47 BGA-G27 RSV19
J28  | 48 BGA-J28 RSV06
H28  | 49 BGA-H28 RSV07
G26  | 50 BGA-G26 RSV21
H26  | 51 BGA-H26 DDRSLRATE1
A14  | 52 BGA-A14 DDRA00
A15  | 53 BGA-A15 DDRA04
B14  | 54 BGA-B14 DDRA01
B15  | 55 BGA-B15 DDRA06
F14  | 56 BGA-F14 DDRA02
F13  | 57 BGA-F13 DDRA03
A13  | 58 BGA-A13 DDRBA0
C15  | 59 BGA-C15 DDRA05
D15  | 60 BGA-D15 DDRA07
F15  | 61 BGA-F15 DDRA08
E15  | 62 BGA-E15 DDRA09
E16  | 63 BGA-E16 DDRA10
D16  | 64 BGA-D16 DDRA11
C16  | 65 BGA-C16 DDRA13
E17  | 66 BGA-E17 DDRA12
D17  | 67 BGA-D17 DDRA14
C17  | 68 BGA-C17 DDRA15
A18  | 69 BGA-A18 DDRCB07
B13  | 70 BGA-B13 DDRBA1
C13  | 71 BGA-C13 DDRBA2
D13  | 72 BGA-D13 DDRODT0
D12  | 73 BGA-D12 DDRCASZ
C12  | 74 BGA-C12 DDRCE1Z
E12  | 75 BGA-E12 DDRWEZ
E19  | 76 BGA-E19 DDRCB00
A20  | 77 BGA-A20 DDRDQM8
D19  | 78 BGA-D19 DDRCB02
C20  | 79 BGA-C20 DDRCB01
B20  | 80 BGA-B20 DDRCB03
B19  | 81 BGA-B19 DDRDQS8N
C19  | 82 BGA-C19 DDRCB04
C18  | 83 BGA-C18 DDRCB05
B18  | 84 BGA-B18 DDRCB06
E18  | 85 BGA-E18 DDRCKE1
C11  | 86 BGA-C11 DDRCE0Z
C10  | 87 BGA-C10 DDRRASZ
D11  | 88 BGA-D11 DDRCKE0
A12  | 89 BGA-A12 DDRCLKOUTP0
E11  | 90 BGA-E11 DDRRESETZ
H29  | 91 BGA-H29 DDRCLKN
G29  | 92 BGA-G29 DDRCLKP
B12  | 93 BGA-B12 DDRCLKOUTN0
B16  | 94 BGA-B16 DDRCLKOUTN1
A16  | 95 BGA-A16 DDRCLKOUTP1
E29  | 96 BGA-E29 DDRDQM0
E28  | 97 BGA-E28 DDRD00
D29  | 98 BGA-D29 DDRD01
D28  | 99 BGA-D28 DDRD03
E27  | 100 BGA-E27 DDRD02
D27  | 101 BGA-D27 DDRD04
B28  | 102 BGA-B28 DDRD05
C27  | 103 BGA-C27 DDRDQM1
E26  | 104 BGA-E26 DDRD06
F25  | 105 BGA-F25 DDRD07
D25  | 106 BGA-D25 DDRD11
F24  | 107 BGA-F24 DDRD08
E25  | 108 BGA-E25 DDRD10
D26  | 109 BGA-D26 DDRD12
E24  | 110 BGA-E24 DDRD09
A27  | 111 BGA-A27 DDRDQS1P
C26  | 112 BGA-C26 DDRD13
B26  | 113 BGA-B26 DDRD14
A25  | 114 BGA-A25 DDRDQM2
A26  | 115 BGA-A26 DDRD15
B27  | 116 BGA-B27 DDRDQS1N
F23  | 117 BGA-F23 DDRD16
F22  | 118 BGA-F22 DDRD17
E23  | 119 BGA-E23 DDRD19
D24  | 120 BGA-D24 DDRD18
B24  | 121 BGA-B24 DDRDQS2N
A23  | 122 BGA-A23 DDRD20
A22  | 123 BGA-A22 DDRDQM3
B23  | 124 BGA-B23 DDRD21
C24  | 125 BGA-C24 DDRD22
E22  | 126 BGA-E22 DDRD23
F20  | 127 BGA-F20 DDRD25
D21  | 128 BGA-D21 DDRD24
E21  | 129 BGA-E21 DDRD26
D22  | 130 BGA-D22 DDRD28
F21  | 131 BGA-F21 DDRD27
C21  | 132 BGA-C21 DDRD29
B22  | 133 BGA-B22 DDRD30
C22  | 134 BGA-C22 DDRD31
B21  | 135 BGA-B21 DDRDQS3N
E10  | 136 BGA-E10 DDRD32
D10  | 137 BGA-D10 DDRD33
A10  | 138 BGA-A10 DDRDQM4
D9   | 139 BGA-D9 DDRD35
B10  | 140 BGA-B10 DDRD34
B9   | 141 BGA-B9 DDRDQS4N
E9   | 142 BGA-E9 DDRD36
C9   | 143 BGA-C9 DDRD37
A8   | 144 BGA-A8 DDRDQM5
B8   | 145 BGA-B8 DDRD38
E8   | 146 BGA-E8 DDRD39
C7   | 147 BGA-C7 DDRD43
A7   | 148 BGA-A7 DDRD40
B7   | 149 BGA-B7 DDRD44
E7   | 150 BGA-E7 DDRD42
D7   | 151 BGA-D7 DDRD41
B6   | 152 BGA-B6 DDRDQS5P
E6   | 153 BGA-E6 DDRD45
D6   | 154 BGA-D6 DDRD46
B5   | 155 BGA-B5 DDRDQM6
C6   | 156 BGA-C6 DDRD47
A6   | 157 BGA-A6 DDRDQS5N
C5   | 158 BGA-C5 DDRD48
A5   | 159 BGA-A5 DDRD49
A4   | 160 BGA-A4 DDRD51
B4   | 161 BGA-B4 DDRD50
D4   | 162 BGA-D4 DDRD52
B2   | 163 BGA-B2 DDRDQM7
E4   | 164 BGA-E4 DDRD53
C4   | 165 BGA-C4 DDRD54
B3   | 166 BGA-B3 DDRDQS6P
C3   | 167 BGA-C3 DDRD55
C2   | 168 BGA-C2 DDRD59
F4   | 169 BGA-F4 DDRD56
E2   | 170 BGA-E2 DDRD58
D2   | 171 BGA-D2 DDRD57
F2   | 172 BGA-F2 DDRD60
F3   | 173 BGA-F3 DDRD61
F1   | 174 BGA-F1 DDRD63
E1   | 175 BGA-E1 DDRD62
H24  | 176 BGA-H24 PTV15
C29  | 177 BGA-C29 DDRDQS0N
C28  | 178 BGA-C28 DDRDQS0P
A24  | 179 BGA-A24 DDRDQS2P
A21  | 180 BGA-A21 DDRDQS3P
A9   | 181 BGA-A9 DDRDQS4P
A3   | 182 BGA-A3 DDRDQS6N
C1   | 183 BGA-C1 DDRDQS7N
D1   | 184 BGA-D1 DDRDQS7P
A19  | 185 BGA-A19 DDRDQS8P
E13  | 186 BGA-E13 DDRODT1
H27  | 187 BGA-H27 DDRSLRATE0
J24  | 188 BGA-J24 RSV08
AD23 | 189 BGA-AD23 DONE
AG23 | 190 BGA-AG23 TIMI1
AC23 | 191 BGA-AC23 RSV03
AE29 | 192 BGA-AE29 EMU00
AF29 | 193 BGA-AF29 EMU01
AE28 | 194 BGA-AE28 EMU02
AF28 | 195 BGA-AF28 EMU03
AE26 | 196 BGA-AE26 EMU04
AD25 | 197 BGA-AD25 EMU05
AE25 | 198 BGA-AE25 EMU07
AF25 | 199 BGA-AF25 EMU06
AF27 | 200 BGA-AF27 EMU08
AF26 | 201 BGA-AF26 EMU10
AG29 | 202 BGA-AG29 EMU09
AG28 | 203 BGA-AG28 EMU11
AG25 | 204 BGA-AG25 EMU13
AG27 | 205 BGA-AG27 EMU12
AH28 | 206 BGA-AH28 EMU14
AJ27 | 207 BGA-AJ27 EMU15
AJ26 | 208 BGA-AJ26 EMU17
AH27 | 209 BGA-AH27 EMU16
AH25 | 210 BGA-AH25 EMU18
AJ25 | 211 BGA-AJ25 RSV01
AE17 | 212 BGA-AE17 EXTFRAMEEVENT
AD18 | 213 BGA-AD18 RESETSTATZ
AF16 | 214 BGA-AF16 MDCLK
AJ20 | 215 BGA-AJ20 GPIO00
AG18 | 216 BGA-AG18 GPIO01
AD19 | 217 BGA-AD19 GPIO02
AE19 | 218 BGA-AE19 GPIO03
AF18 | 219 BGA-AF18 GPIO04
AD21 | 220 BGA-AD21 GPIO15
AE18 | 221 BGA-AE18 GPIO05
AG20 | 222 BGA-AG20 GPIO06
AH19 | 223 BGA-AH19 GPIO07
AE21 | 224 BGA-AE21 GPIO09
AJ19 | 225 BGA-AJ19 GPIO08
AD20 | 226 BGA-AD20 GPIO11
AE20 | 227 BGA-AE20 GPIO12
AH20 | 228 BGA-AH20 GPIO14
AE22 | 229 BGA-AE22 LRESETZ
AF21 | 230 BGA-AF21 GPIO13
AC19 | 231 BGA-AC19 PORZ
AC20 | 232 BGA-AC20 LRESETNMIENZ
AC25 | 233 BGA-AC25 NMIZ
AD22 | 234 BGA-AD22 RSV12
V4   | 235 BGA-V4 RSV14
T5   | 236 BGA-T5 MCMTXN0
R5   | 237 BGA-R5 MCMTXP0
W2   | 238 BGA-W2 MCMCLKN
W1   | 239 BGA-W1 MCMCLKP
V2   | 240 BGA-V2 MCMREFCLKOUTP
V1   | 241 BGA-V1 MCMREFCLKOUTN
V3   | 242 BGA-V3 MCMRXFLCLK
W3   | 243 BGA-W3 MCMRXFLDAT
AA3  | 244 BGA-AA3 MCMRXPMCLK
T2   | 245 BGA-T2 MCMRXN0
R2   | 246 BGA-R2 MCMRXP0
P1   | 247 BGA-P1 MCMRXN1
R1   | 248 BGA-R1 MCMRXP1
N2   | 249 BGA-N2 MCMRXN3
L1   | 250 BGA-L1 MCMRXN2
M1   | 251 BGA-M1 MCMRXP2
M4   | 252 BGA-M4 MCMTXP2
M2   | 253 BGA-M2 MCMRXP3
R4   | 254 BGA-R4 MCMTXN1
P4   | 255 BGA-P4 MCMTXP1
Y3   | 256 BGA-Y3 MCMRXPMDAT
AA2  | 257 BGA-AA2 MCMTXPMCLK
Y1   | 258 BGA-Y1 MCMTXFLCLK
Y2   | 259 BGA-Y2 MCMTXFLDAT
AA1  | 260 BGA-AA1 MCMTXPMDAT
L4   | 261 BGA-L4 MCMTXN2
N5   | 262 BGA-N5 MCMTXP3
M5   | 263 BGA-M5 MCMTXN3
AG16 | 264 BGA-AG16 MDIO
AF24 | 265 BGA-AF24 UARTRXD
AH23 | 266 BGA-AH23 TIMO0
AC24 | 267 BGA-AC24 RESETZ
AD16 | 268 BGA-AD16 RSV23
AH22 | 269 BGA-AH22 SPISOMI
AE16 | 270 BGA-AE16 RSV22
AF17 | 271 BGA-AF17 RSV25
AG17 | 272 BGA-AG17 RSV24
AH18 | 273 BGA-AH18 PASSCLKN
AJ18 | 274 BGA-AJ18 PASSCLKP
AH17 | 275 BGA-AH17 PCIECLKP
AE14 | 276 BGA-AE14 RSV16
AG14 | 277 BGA-AG14 PCIETXN0
AG13 | 278 BGA-AG13 PCIETXP0
AJ17 | 279 BGA-AJ17 PCIECLKN
AH16 | 280 BGA-AH16 SRIOSGMIICLKN
AJ14 | 281 BGA-AJ14 PCIERXN0
AJ13 | 282 BGA-AJ13 PCIERXP0
AH13 | 283 BGA-AH13 PCIERXP1
AH12 | 284 BGA-AH12 PCIERXN1
AF13 | 285 BGA-AF13 PCIETXP1
AF12 | 286 BGA-AF12 PCIETXN1
AJ11 | 287 BGA-AJ11 RIORXN0
AB27 | 288 BGA-AB27 PHYSYNC
J25  | 289 BGA-J25 RSV09
AC22 | 290 BGA-AC22 RSV13
AE8  | 291 BGA-AE8 RSV15
AF6  | 292 BGA-AF6 RIOTXN3
AF7  | 293 BGA-AF7 RIOTXP3
AJ10 | 294 BGA-AJ10 RIORXP0
AH10 | 295 BGA-AH10 RIORXN1
AH9  | 296 BGA-AH9 RIORXP1
AF10 | 297 BGA-AF10 RIOTXP1
AJ7  | 298 BGA-AJ7 RIORXN2
AJ8  | 299 BGA-AJ8 RIORXP2
AH7  | 300 BGA-AH7 RIORXP3
AH6  | 301 BGA-AH6 RIORXN3
AG8  | 302 BGA-AG8 RIOTXP2
AF9  | 303 BGA-AF9 RIOTXN1
AG11 | 304 BGA-AG11 RIOTXN0
AG10 | 305 BGA-AG10 RIOTXP0
AG7  | 306 BGA-AG7 RIOTXN2
AA28 | 307 BGA-AA28 RP1CLKN
Y29  | 308 BGA-Y29 RP1FBP
AA29 | 309 BGA-AA29 RP1FBN
AE5  | 310 BGA-AE5 RSV17
AF3  | 311 BGA-AF3 SGMIITXN0
AF4  | 312 BGA-AF4 SGMIITXP0
AH3  | 313 BGA-AH3 SGMIIRXN0
AH4  | 314 BGA-AH4 SGMIIRXP0
AJ4  | 315 BGA-AJ4 SGMIIRXN1
AJ5  | 316 BGA-AJ5 SGMIIRXP1
AG5  | 317 BGA-AG5 SGMIITXP1
AG4  | 318 BGA-AG4 SGMIITXN1
AG21 | 319 BGA-AG21 SPICLK
AJ21 | 320 BGA-AJ21 SPISIMO
AH21 | 321 BGA-AH21 SPISCS0
AH24 | 322 BGA-AH24 UARTCTS
AJ22 | 323 BGA-AJ22 SPISCS1
AJ16 | 324 BGA-AJ16 SRIOSGMIICLKP
AC29 | 325 BGA-AC29 SYSCLKP
AD29 | 326 BGA-AD29 TCK
AD28 | 327 BGA-AD28 TDI
AC27 | 328 BGA-AC27 TDO
AC26 | 329 BGA-AC26 TMS
H23  | 330 BGA-H23 RSV10
J23  | 331 BGA-J23 RSV11
AJ23 | 332 BGA-AJ23 TIMI0
AF23 | 333 BGA-AF23 TIMO1
AD26 | 334 BGA-AD26 TRSTZ
AG24 | 335 BGA-AG24 UARTRTS
AJ24 | 336 BGA-AJ24 UARTTXD
[Model Data]
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[End Model Data]
[End Package Model]
|   Model Cell s_ICLKRX10G_0p9
|s_iclkrx10g_0p9  [08July11 revision 1.3]
[Model]   s_iclkrx10g_0p9
Model_type   Series
Polarity   Non-Inverting
|Vinl =  1.15
|Vinh =  1.25
C_comp   0.01p   0.01p   0.01p
[Temperature Range]   25   125   -40
[Voltage Range]   0.9   0.81   0.99
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|   Model Cell s_ICLKRX10G_1
|s_iclkrx10g_1  [08July11 revision 1.3]
[Model]   s_iclkrx10g_1
Model_type   Series
C_comp   0.01p   0.01p   0.01p
[Voltage Range]   1   0.9   1.1
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|   Model Cell s_ilvds18g_5P
|ilvds18g_5P
[Model]   s_ilvds18g_5P
Model_type   Series
C_comp   0.01p   0.01p   0.01p
[Voltage Range]   1.8 1.71 1.89
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| Models and submodels in the file (153): bi2c18gfz (I/O_open_drain), iclkrx10g_0p9 (Input), s_iclkrx10g_0p9 (Series), iclkrx10g_1 (Input), s_iclkrx10g_1 (Series), ihhv18g (Input), ilvds18g_5P (Input), s_ilvds18g_5P (Series), ocml10g_0p9 (Output), ocml10g_1 (Output), BC1840DGHYPBFB_WK_PD (Input), BC1840DGHYPBFB_WK_PU (Input), BC1840DGHYPBFB_DRIVER_MODE (I/O), BC1850CGHYPBFB_WK_PD (Input), BC1850CGHYPBFB_WK_PU (Input), BC1850CGHYPBFB_DRIVER_MODE (I/O), CSCDVG_SLOWEST_8MA_NT (I/O), CSCDVG_SLOWEST_8MA_HT8MA (I/O), CSCDVG_SLOWEST_8MA_FT8MA (I/O), CSCDVG_SLOWEST_9MA_NT (I/O), CSCDVG_SLOWEST_9MA_HT9MA (I/O), CSCDVG_SLOWEST_9MA_FT9MA (I/O), CSCDVG_SLOWEST_10MA_NT (I/O), CSCDVG_SLOWEST_10MA_HT10MA (I/O), CSCDVG_SLOWEST_10MA_FT10MA (I/O), CSCDVG_SLOW_8MA_NT (I/O), CSCDVG_SLOW_8MA_HT8MA (I/O), CSCDVG_SLOW_8MA_FT8MA (I/O), CSCDVG_SLOW_9MA_NT (I/O), CSCDVG_SLOW_9MA_HT9MA (I/O), CSCDVG_SLOW_9MA_FT9MA (I/O), CSCDVG_SLOW_10MA_NT (I/O), CSCDVG_SLOW_10MA_HT10MA (I/O), CSCDVG_SLOW_10MA_FT10MA (I/O), CSCDVG_FAST_8MA_NT (I/O), CSCDVG_FAST_8MA_HT8MA (I/O), CSCDVG_FAST_8MA_FT8MA (I/O), CSCDVG_FAST_9MA_NT (I/O), CSCDVG_FAST_9MA_HT9MA (I/O), CSCDVG_FAST_9MA_FT9MA (I/O), CSCDVG_FAST_10MA_NT (I/O), CSCDVG_FAST_10MA_HT10MA (I/O), CSCDVG_FAST_10MA_FT10MA (I/O), CSCDVG_FASTEST_8MA_NT (I/O), CSCDVG_FASTEST_8MA_HT8MA (I/O), CSCDVG_FASTEST_8MA_FT8MA (I/O), CSCDVG_FASTEST_9MA_NT (I/O), CSCDVG_FASTEST_9MA_HT9MA (I/O), CSCDVG_FASTEST_9MA_FT9MA (I/O), CSCDVG_FASTEST_10MA_NT (I/O), CSCDVG_FASTEST_10MA_HT10MA (I/O), CSCDVG_FASTEST_10MA_FT10MA (I/O), DIFF_FT_TH_8MA (Dynamic_clamp), DIFF_HT_TH_9MA (Dynamic_clamp), DIFF_NT (Dynamic_clamp), DIFF_HT_TH_8MA (Dynamic_clamp), DIFF_FT_TH_10MA (Dynamic_clamp), DIFF_FT_TH_9MA (Dynamic_clamp), DIFF_HT_TH_10MA (Dynamic_clamp), CSCDDVG_SLOWEST_8MA_FT8MA_N (I/O), CSCDDVG_SLOWEST_8MA_HT8MA_N (I/O), CSCDDVG_SLOWEST_8MA_NT_N (I/O), CSCDDVG_SLOW_8MA_NT_N (I/O), CSCDDVG_SLOW_8MA_FT8MA_N (I/O), CSCDDVG_SLOW_8MA_HT8MA_N (I/O), CSCDDVG_FAST_8MA_NT_N (I/O), CSCDDVG_FAST_8MA_FT8MA_N (I/O), CSCDDVG_FAST_8MA_HT8MA_N (I/O), CSCDDVG_FASTEST_8MA_FT8MA_N (I/O), CSCDDVG_FASTEST_8MA_HT8MA_N (I/O), CSCDDVG_FASTEST_8MA_NT_N (I/O), CSCDDVG_SLOWEST_10MA_NT_N (I/O), CSCDDVG_SLOWEST_10MA_FT10MA_N (I/O), CSCDDVG_SLOWEST_10MA_HT10MA_N (I/O), CSCDDVG_SLOW_10MA_FT10MA_N (I/O), CSCDDVG_SLOW_10MA_NT_N (I/O), CSCDDVG_SLOW_10MA_HT10MA_N (I/O), CSCDDVG_FAST_10MA_FT10MA_N (I/O), CSCDDVG_FAST_10MA_NT_N (I/O), CSCDDVG_FAST_10MA_HT10MA_N (I/O)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
